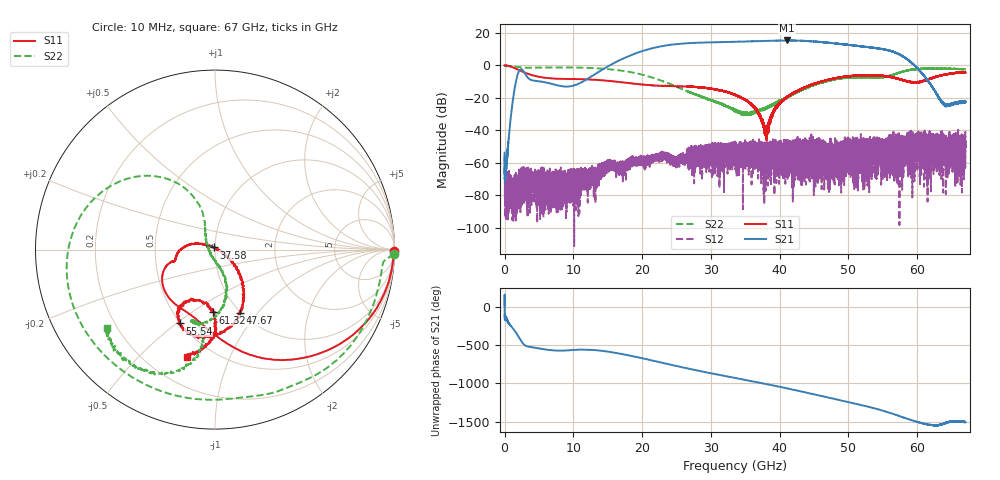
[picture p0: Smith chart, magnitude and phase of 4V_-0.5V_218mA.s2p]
! MARKI MICROWAVE INC.
! Date:  10/21/2020
! Model Number:  AMM-7210CH
! Description:  2-port Small Signal S-parameter data for AMM-7210CH
! Frequency Range:  10 MHz to 67 GHz
! Port Configuration:  PORT 1: Input
!  PORT 2: Output
! Bias Condition: Vd = +4.0V, Vg = -0.5V
! AMM-7210CH s2p files are only valid for small signal conditions (below -10 dBm input power)
# Hz S  dB  R 50
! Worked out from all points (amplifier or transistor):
!   20001 points, 10 MHz to 67 GHz, reference 50 ohm
!   highest |S21| = 15.2 dB at 41.06 GHz (marker M1)
!   |S21| within 3 dB of that: 23.59 GHz to 50.53 GHz (26.94 GHz wide, 72.7 % of centre)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
!   unconditionally stable (mu >= 1): start of sweep to 17.07 MHz; 22.71 MHz to end of sweep
!   at 11.17 GHz: K = 1174.31, MAG = -4.6 dB, |S12| = -68.8 dB
!   at 33.51 GHz: K = 39.07, MAG = 14.5 dB, |S12| = -52.4 dB
!   at 67 GHz: K = 771.13, MAG = -16.8 dB, |S12| = -52.5 dB
!   S11 on the Smith chart (normalised r, x): 10 MHz: open; 37.58 GHz: 0.98, +0.02; 47.67 GHz: 0.99, -0.81; 55.54 GHz: 0.49, -0.51; 61.32 GHz: 0.77, -0.61; 67 GHz: 0.38, -0.69
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1e7  -0.02 -0.6  -53.74 25.4  -59.68 -148.9  -0.02 -1.5
2.254165e9  -3.29 -63.2  -2.72 -62.2  -66.17 -37.9  -1.23 -62.5
1.117723e10  -8.59 -133.0  -10.54 162.3  -70.85 162.4  -1.52 -168.7
1.705896e10  -10.49 -159.4  3.70 104.7  -63.81 125.3  -3.40 148.0
1.994622e10  -11.83 -164.0  8.56 51.1  -58.48 129.0  -5.75 128.0
2.234112e10  -12.61 -164.3  11.25 2.4  -55.36 107.8  -8.82 114.9
2.458528e10  -12.88 -166.2  12.75 -43.7  -57.35 85.7  -12.44 108.6
2.753954e10  -13.25 -171.5  13.70 -101.5  -51.94 95.5  -17.73 115.1
3.068472e10  -14.92 177.2  14.11 -158.8  -62.02 82.1  -22.72 133.7
3.3505e10  -18.12 165.1  14.39 151.9  -52.40 43.8  -27.46 159.3
3.758469e10  -37.06 122.2  14.90 80.2  -51.43 -50.2  -26.56 -108.5
4.106147e10  -19.77 -36.1  15.20 15.5  -49.75 -147.8  -19.72 -75.5
4.277977e10  -15.37 -42.6  15.08 -18.5  -52.75 -108.4  -16.17 -70.3
4.467223e10  -11.97 -51.5  14.73 -56.4  -47.78 -170.3  -12.77 -75.1
4.767004e10  -8.45 -68.8  13.58 -116.6  -52.71 -138.4  -8.86 -87.3
5.114012e10  -6.30 -90.8  11.99 173.3  -54.06 0.3  -7.44 -103.6
5.356181e10  -6.20 -105.8  10.72 119.4  -49.29 -62.0  -7.74 -107.1
5.553801e10  -6.81 -115.6  9.44 68.5  -49.74 47.6  -6.99 -100.5
5.583612e10  -7.02 -116.9  9.08 60.0  -63.11 -113.0  -6.64 -99.6
5.852576e10  -9.85 -116.4  3.75 -22.0  -41.47 172.2  -3.23 -105.4
6.13159e10  -9.11 -91.9  -8.28 -93.1  -54.14 124.5  -2.10 -122.0
6.7e10  -4.41 -105.7  -22.26 -63.3  -52.49 -148.7  -2.54 -144.0
